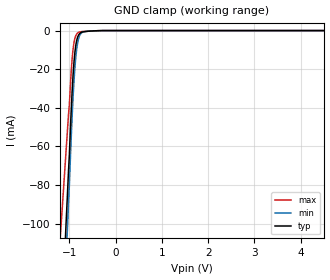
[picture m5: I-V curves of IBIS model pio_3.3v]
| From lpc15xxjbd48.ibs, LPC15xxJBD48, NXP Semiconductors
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[Model] pio_3.3v
Model_type Input
Vinl = 990.000mV
Vinh = 2.31000V
C_comp 598.000fF 598.000fF 598.000fF
| variable typ   min   max
[Voltage Range] 3.30000V 3.00000V 3.60000V
[POWER Clamp Reference] 3.30000V 3.00000V 3.60000V
[GND Clamp Reference] 0.00000V 0.00000V 0.00000V
[Temperature Range]   25   85   -40
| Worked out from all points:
|   GND clamp passes 1 mA (typ) near -0.75 V on its own axis
[GND Clamp]
-3.3V     -1.253A    -1.386A    -859.3mA
-1.02V    -73.18mA   -90.22mA   -43.77mA
-1V       -64.02mA   -79.69mA   -38.01mA
-960mV    -40.88mA   -55.21mA   -20.83mA
-940mV    -31.05mA   -44.18mA   -14.35mA
-900mV    -16.12mA   -25.91mA   -6.109mA
-860mV    -7.423mA   -13.38mA   -2.525mA
-840mV    -4.92mA    -9.183mA   -1.69mA
-800mV    -2.24mA    -4.06mA    -902.3uA
-700mV    -656.7uA   -685.1uA   -442.1uA
-280mV    0A         0A         0A
6.6V      0A         0A         0A
[Power Clamp]
-3.3V     0A         0A         0A
0V        0A         0A         0A
3.3V      0A         0A         0A
6.6V      0A         0A         0A
